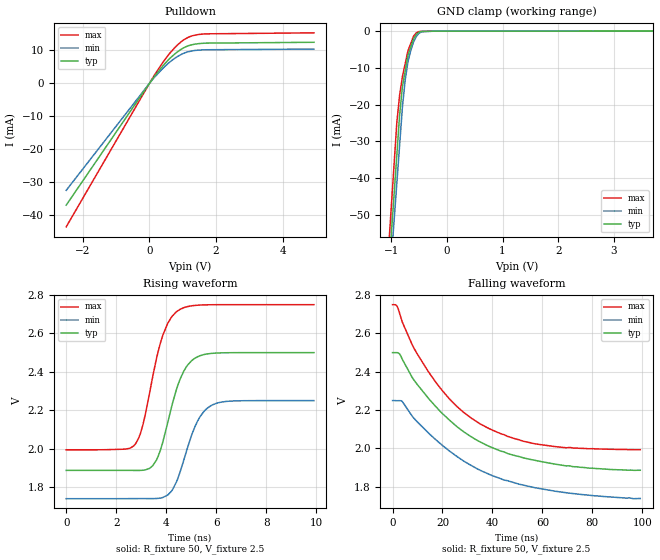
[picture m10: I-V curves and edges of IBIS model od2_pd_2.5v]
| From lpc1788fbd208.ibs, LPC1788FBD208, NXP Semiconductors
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[Model]   od2_pd_2.5v
Model_type I/O_open_drain
Vinl=7.500E-01
Vinh=1.750E+00
Vref=2.500E+00
Rref=2.000E+03
Cref=0.000E+00
Vmeas=1.250E+00
C_comp   5.160E-13   4.910E-13   5.420E-13
[Voltage Range]   2.500E+00   2.250E+00   2.750E+00
[POWER Clamp Reference]   2.500E+00   2.250E+00   2.750E+00
[GND Clamp Reference]   0.000E+00   0.000E+00   0.000E+00
[Pullup Reference]   2.500E+00   2.250E+00   2.750E+00
[Pulldown Reference]   0.000E+00   0.000E+00   0.000E+00
[Temperature Range]   25   85   -40
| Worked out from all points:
|   slope of the pulldown table from 0 to 0.375 V, typ, clamps not added: 75.7 ohm
|   GND clamp passes 1 mA (typ) near -0.55 V on its own axis
|   rising waveform, R_fixture 50, V_fixture 2.5: 20-80 % time 802ps typ, 818ps min, 783ps max; typ from 1.89 V to 2.5 V
|   falling waveform, R_fixture 50, V_fixture 2.5: 20-80 % time 31.4ns typ, 34.3ns min, 27.2ns max; typ from 2.5 V to 1.89 V
[GND Clamp]
-2.5V     -381.4mA   -371.5mA   -393.2mA
-900mV    -33.63mA   -41.3mA    -24.8mA
-850mV    -22.77mA   -30.98mA   -17.38mA
-800mV    -15.14mA   -20.67mA   -12.36mA
-750mV    -10.83mA   -13.28mA   -8.858mA
-700mV    -6.525mA   -8.291mA   -5.352mA
-650mV    -4.333mA   -5.277mA   -3.365mA
-600mV    -2.14mA    -2.967mA   -1.379mA
-550mV    -873.5uA   -1.422mA   -434.8uA
-450mV    -57.55uA   -158uA     -76.16uA
-225mV    -9.459uA   -6.37uA    -2.898uA
5V        20uA       33.33uA    12.5uA
[Pulldown]
-2.5V     -37.02mA   -32.52mA   -43.62mA
152.9mV   2.149mA    1.866mA    2.564mA
591.7mV   7.38mA     6.328mA    8.925mA
771.2mV   9.017mA    7.692mA    10.96mA
970.7mV   10.47mA    8.879mA    12.79mA
1.27V     11.72mA    9.839mA    14.4mA
1.629V    12.19mA    10.19mA    15.01mA
4.94V     12.49mA    10.42mA    15.36mA
[Rising Waveform]
R_fixture = 50
V_fixture = 2.5
V_fixture_min = 2.25
V_fixture_max = 2.75
0s        1.887V     1.739V     1.994V
2.376ns   1.887V     1.739V     1.998V
2.772ns   1.886V     1.74V      2.025V
3.069ns   1.887V     1.74V      2.126V
3.6ns     1.939V     1.74V      2.465V
4.059ns   2.137V     1.758V     2.653V
4.555ns   2.363V     1.879V     2.726V
5.148ns   2.471V     2.116V     2.746V
5.8ns     2.496V     2.225V     2.75V
9.901ns   2.5V       2.25V      2.75V
[Falling Waveform]
R_fixture = 50
V_fixture = 2.5
V_fixture_min = 2.25
V_fixture_max = 2.75
0s        2.5V       2.25V      2.75V
1.798ns   2.5V       2.249V     2.743V
3.896ns   2.465V     2.245V     2.66V
8.591ns   2.357V     2.157V     2.523V
17.28ns   2.219V     2.046V     2.346V
25.77ns   2.114V     1.958V     2.219V
35.07ns   2.034V     1.887V     2.128V
46.15ns   1.973V     1.832V     2.063V
58.04ns   1.935V     1.793V     2.022V
99.2ns    1.887V     1.739V     1.994V
[Ramp]
dV/dt_r   3.6807E-01/7.9470E-10   3.0650E-01/8.1600E-10   4.5371E-01/7.7670E-10
dV/dt_f   3.6807E-01/3.1494E-08   3.0650E-01/3.4327E-08   4.5371E-01/2.7399E-08
R_load = 50
